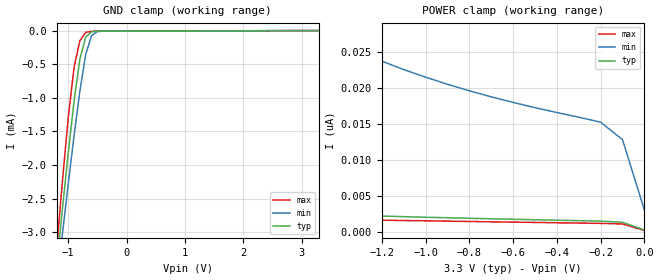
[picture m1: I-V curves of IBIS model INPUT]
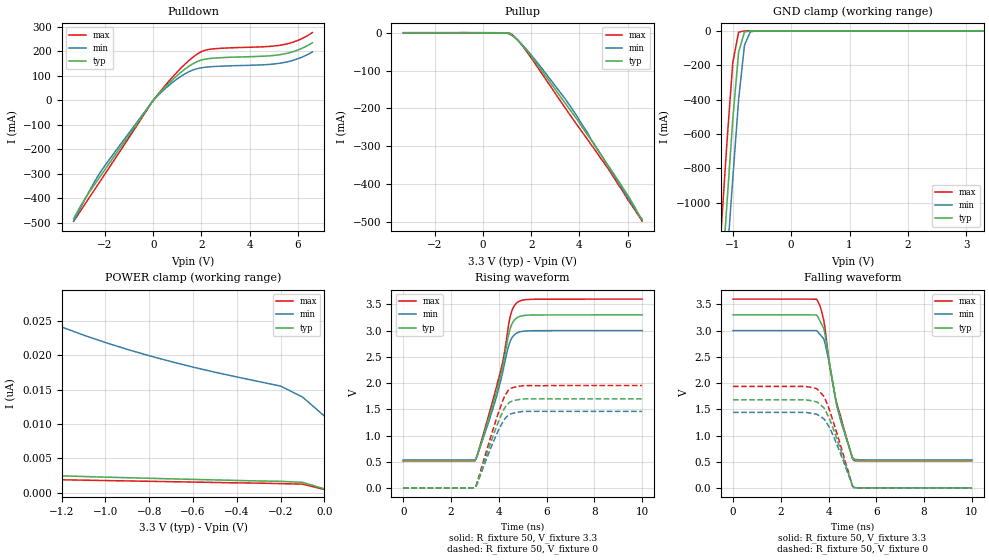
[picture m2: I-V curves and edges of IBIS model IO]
|   PERICOM SEMICONDUCTOR CORP
|   IBIS Model of PI4ULS3V204
|   Product Family: ULS
|   TSSOP-14 (L) Package
[IBIS Ver] 3.2
[Comment char] |_char
[File Name] pi4uls3v204_l_33v.ibs
[File Rev] 1.0
[Source] File originated at Pericom Semiconductor Corp.
[Date] 09/01/2017
[Disclaimer] (C) Copyright PERICOM Semiconductor Corporation
   All rights reserved
  Pericom Semiconductor Corporation hereby grants the user of
  this IBIS model a non-exclusive, nontransferable license to
  use this IBIS model under the following terms.
  This IBIS model is provided on an "AS IS" basis and Pericom
  makes absolutely no warranty with respect to the information
  contained herein. PERICOM DISCLAIMS AND CUSTOMER WAIVES ALL
  WARRANTIES, EXPRESSED OR IMPLIED, INCLUDING WARRANTIES OF
  MERCHANTABILITY OR FITNESS FOR A PARTICULAR PURPOSE. The
  entire risk as to quality and performance is with the customer.
  Accordingly, in no event shall the company be liable for any
  damages, whether in contract or tort, including any lost
  profits or other incidental, consequential, exemplary, or
  punitive damages arising out of the use or application of the
  IBIS model provided in this package. Further, Pericom reserves
  the right to make changes without notice to any product herein
  to improve reliability, function, or design. Pericom does not
  convey any license under patent rights or any other intellectual
  property rights, including those of third parties.
  The user is granted this license only to use the IBIS model
  and is not granted rights to sell, load, rent, lease or license
  the IBIS model in whole or in part, or in modified form to anyone
  other than user. User may modify the IBIS model to suit its specific
  application but rights to derivative works and such modifications
  shall belong to Pericom.
  Pericom is not obligated to provide maintenance or support
  for the licensed IBIS model.
  Contact Pericom at ATTN: APPLICATION ENGINEERING / IBIS MODELS
  1545 Barber Lane Milpitas, CA 95035 USA.
[Component] PI4ULS3V204
[Manufacturer] Pericom Semiconductor Corp.
[Package]
| variable   typ   min   max
R_pkg   0.04200   0.03995   0.04405
L_pkg   2.30669n   2.21200n   2.40138n
C_pkg   0.21108p   0.20715p   0.21500p
[Pin] signal_name  model_name   R_pin   L_pin   C_pin
1   VCCA   POWER   0.03604  2.91900n  0.20300p
2   A1   IO   0.03631  2.73467n  0.19100p
3   A2   IO   0.03658  2.55033n  0.17900p
4   A3   IO   0.03686  2.36600n  0.16700p
5   A4   IO   0.03658  2.55033n  0.17900p
6   NC   NC   0.03631  2.73467n  0.19100p
7   GND   GND   0.03604  2.91900n  0.20300p
8   EN   INPUT   0.03604  2.91900n  0.20300p
9   NC   NC   0.03631  2.73467n  0.19100p
10   B4   IO   0.03658  2.55033n  0.17900p
11   B3   IO   0.03686  2.36600n  0.16700p
12   B2   IO   0.03658  2.55033n  0.17900p
13   B1   IO   0.03631  2.73467n  0.19100p
14   VCCB   POWER   0.03604  2.91900n  0.20300p
| Models and submodels in the file (2): INPUT (Input), IO (I/O)
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[Model] INPUT
Model_type Input
Vinl = 990mV
Vinh = 2.31V
| variable   typ   min   max
C_comp   0.220pF   0.210pF   0.230pF
[Voltage Range]   3.3000V   3.0000V   3.6000V
[POWER Clamp Reference] 3.3000V   3.0000V   3.6000V
[GND Clamp Reference]   0.0000V   0.0000V   0.0000V
[Temperature Range]   25   85   -40
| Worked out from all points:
|   GND clamp passes 1 mA (typ) near -0.89 V on its own axis
[GND Clamp]
| Voltage   I(typ)   I(min)   I(max)
-3.3V     -22.41mA   -20.33mA   -26.05mA
-1.2V     -3.522mA   -3.797mA   -3.269mA
-1.1V     -2.66mA    -3.034mA   -2.25mA
-1V       -1.827mA   -2.286mA   -1.301mA
-900mV    -1.052mA   -1.566mA   -548.2uA
-800mV    -423.5uA   -899.4uA   -150.4uA
-700mV    -98.47uA   -356.4uA   -26.64uA
-600mV    -18.3uA    -75.45uA   -9.991uA
-500mV    -9.6uA     -15.14uA   -8.807uA
3.3V      523pA      908.7pA    22.89pA
[POWER Clamp]
| Voltage   I(typ)   I(min)   I(max)
-3.3V     5.713nA    96.31nA    2.631nA
-3V       4.875nA    76.7nA     2.482nA
-2.6V     4nA        57.04nA    2.307nA
-2V       3.059nA    37.7nA     2.036nA
-1.5V     2.511nA    27.85nA    1.811nA
-1.4V     2.413nA    26.35nA    1.757nA
-1.2V     2.242nA    23.72nA    1.672nA
-900mV    2.009nA    20.52nA    1.536nA
-600mV    1.797nA    18nA       1.403nA
-200mV    1.539nA    15.26nA    1.225nA
-100mV    1.373nA    12.84nA    1.148nA
0V        314.4pA    3.086nA    253.5pA
[Model]   IO
Model_type I/O
Vinl=0.15
Vinh=3.2
Enable   Active-High
Vref =   3.3
Rref =   50
Cref =   15p
Vmeas =   1.65
| variable   typ   min   max
C_comp   3.620E-12   3.610E-12   3.630E-12
[Voltage Range]   3.3000V   3.0000V   3.6000V
[POWER Clamp Reference] 3.3000V   3.0000V   3.6000V
[GND Clamp Reference]   0.000E+00   0.000E+00   0.000E+00
[Pullup Reference]   3.3000V   3.0000V   3.6000V
[Pulldown Reference]   0.000E+00   0.000E+00   0.000E+00
[Temperature Range]   25   85   -40
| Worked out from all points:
|   slope of the pulldown table from 0 to 0.495 V, typ, clamps not added: 9.25 ohm
|   slope of the pullup table from 0 to 0.495 V, typ, clamps not added: 10.1 kohm
|   GND clamp passes 1 mA (typ) near -0.71 V on its own axis
|   rising waveform, R_fixture 50, V_fixture 3.3: 20-80 % time 925ps typ, 900ps min, 951ps max; typ from 0.525 V to 3.3 V
|   falling waveform, R_fixture 50, V_fixture 3.3: 20-80 % time 745ps typ, 711ps min, 775ps max; typ from 3.3 V to 0.526 V
|   rising waveform, R_fixture 50, V_fixture 0: 20-80 % time 799ps typ, 793ps min, 804ps max; typ from 0.002 V to 1.7 V
|   falling waveform, R_fixture 50, V_fixture 0: 20-80 % time 778ps typ, 764ps min, 792ps max; typ from 1.68 V to 0.002 V
[GND Clamp]
| Voltage   I(typ)   I(min)   I(max)
-3.3V     -11.83A    -11.71A    -12A
-1.2V     -1.497A    -1.804A    -1.164A
-1.1V     -1.005A    -1.332A    -648.2mA
-1V       -514.4mA   -860.5mA   -184.8mA
-900mV    -123.7mA   -400mA     -7.522mA
-800mV    -6.738mA   -83.76mA   -632.8uA
-700mV    -436.7uA   -5.934mA   -74.67uA
-500mV    -2.716uA   -28.54uA   -128.4nA
3.3V      551pA      16.17nA    48.7pA
[POWER Clamp]
| Voltage   I(typ)   I(min)   I(max)
-3.3V     6.13nA     97.23nA    3.05nA
-2.9V     5.016nA    71.95nA    2.82nA
-2.5V     4.152nA    53.75nA    2.602nA
-2V       3.338nA    38.26nA    2.314nA
-1.5V     2.736nA    28.28nA    2.045nA
-1.3V     2.536nA    25.37nA    1.928nA
-1.2V     2.438nA    24.1nA     1.867nA
-900mV    2.174nA    20.84nA    1.706nA
-600mV    1.925nA    18.27nA    1.536nA
-200mV    1.643nA    15.51nA    1.312nA
-100mV    1.503nA    13.92nA    1.238nA
0V        551.5pA    11.15nA    457.6pA
[Pullup]
| Voltage   I(typ)   I(min)   I(max)
-3.3V     39.21uA    25.56uA    63.93uA
900mV     -121.2uA   -241.9uA   -91.96uA
1.2V      -5.901mA   -7.186mA   -4.522mA
1.5V      -23.27mA   -23.22mA   -23.69mA
1.9V      -53.74mA   -50.92mA   -57.44mA
3.4V      -185.2mA   -173.8mA   -197.6mA
3.9V      -228.6mA   -220.1mA   -243.1mA
4.4V      -275.2mA   -270.5mA   -287.5mA
4.5V      -284.6mA   -283.7mA   -296.9mA
5.3V      -360mA     -363.9mA   -369.6mA
6.1V      -438.5mA   -444.6mA   -448.8mA
6.6V      -494.6mA   -492.2mA   -497.8mA
[Pulldown]
| Voltage   I(typ)   I(min)   I(max)
-3.3V     -484.4mA   -494.4mA   -495mA
-2.8V     -398mA     -399.2mA   -420.5mA
-2.2V     -311.6mA   -295.7mA   -331mA
0V        -223.3pA   -2.732nA   -109.7pA
900mV     92.81mA    80.52mA    105.6mA
1.3V      126.1mA    107mA      146mA
1.7V      152.1mA    125.5mA    180.1mA
2V        164.5mA    132.8mA    198.9mA
2.4V      171.2mA    137.1mA    209.1mA
5.2V      185.6mA    150.7mA    224.1mA
5.9V      201.9mA    166.4mA    241.1mA
6.6V      235.2mA    197.5mA    276.8mA
[Rising Waveform]
R_fixture = 50
V_fixture = 3.3
V_fixture_min = 3.0
V_fixture_max = 3.6
| Time   V(typ)   V(min)   V(max)
0s        524.6mV    533.9mV    514.8mV
3ns       524.6mV    533.9mV    514.8mV
3.65ns    1.439V     1.368V     1.51V
4.05ns    2.097V     1.996V     2.188V
4.2ns     2.405V     2.291V     2.494V
4.45ns    2.999V     2.766V     3.214V
4.6ns     3.17V      2.896V     3.436V
4.8ns     3.256V     2.964V     3.546V
5.4ns     3.297V     2.997V     3.597V
10ns      3.3V       3V         3.6V
[Falling Waveform]
R_fixture = 50
V_fixture = 3.3
V_fixture_min = 3.0
V_fixture_max = 3.6
| Time   V(typ)   V(min)   V(max)
0s        3.3V       3V         3.6V
3.5ns     3.3V       3V         3.6V
3.65ns    3.175V     2.923V     3.462V
3.8ns     3.041V     2.84V      3.198V
4.05ns    2.355V     2.345V     2.305V
4.3ns     1.673V     1.679V     1.695V
4.55ns    1.251V     1.216V     1.287V
5ns       577.2mV    589.5mV    563mV
5.05ns    541.7mV    555mV      527.3mV
10ns      525.7mV    536mV      515.3mV
[Rising Waveform]
R_fixture = 50
V_fixture = 0
V_fixture_min = 0
V_fixture_max = 0
| Time   V(typ)   V(min)   V(max)
0s        2.461mV    2.455mV    2.457mV
3ns       2.461mV    2.455mV    2.457mV
3.1ns     103.2mV    88.8mV     118.1mV
3.75ns    982mV      859.8mV    1.105V
4.1ns     1.389V     1.201V     1.586V
4.25ns    1.53V      1.316V     1.756V
4.4ns     1.611V     1.381V     1.866V
4.5ns     1.646V     1.412V     1.898V
5.05ns    1.698V     1.46V      1.952V
10ns      1.699V     1.46V      1.953V
[Falling Waveform]
R_fixture = 50
V_fixture = 0
V_fixture_min = 0
V_fixture_max = 0
| Time   V(typ)   V(min)   V(max)
0s        1.681V     1.441V     1.936V
3ns       1.681V     1.441V     1.936V
3.5ns     1.642V     1.405V     1.895V
3.8ns     1.531V     1.321V     1.751V
3.85ns    1.495V     1.291V     1.707V
4.05ns    1.306V     1.144V     1.471V
4.45ns    799.9mV    712.8mV    891.2mV
5ns       43.37mV    43.05mV    43.51mV
5.05ns    11.77mV    13.67mV    14.42mV
10ns      2.47mV     2.466mV    2.456mV
[Ramp]
| variable   typ   min   max
dV/dt_r   1.0178E+00/7.9959E-10  8.7492E-01/7.9368E-10  1.1707E+00/8.0441E-10
dV/dt_f   1.6645E+00/7.4438E-10  1.4783E+00/7.1075E-10  1.8508E+00/7.7533E-10
R_load = 50
